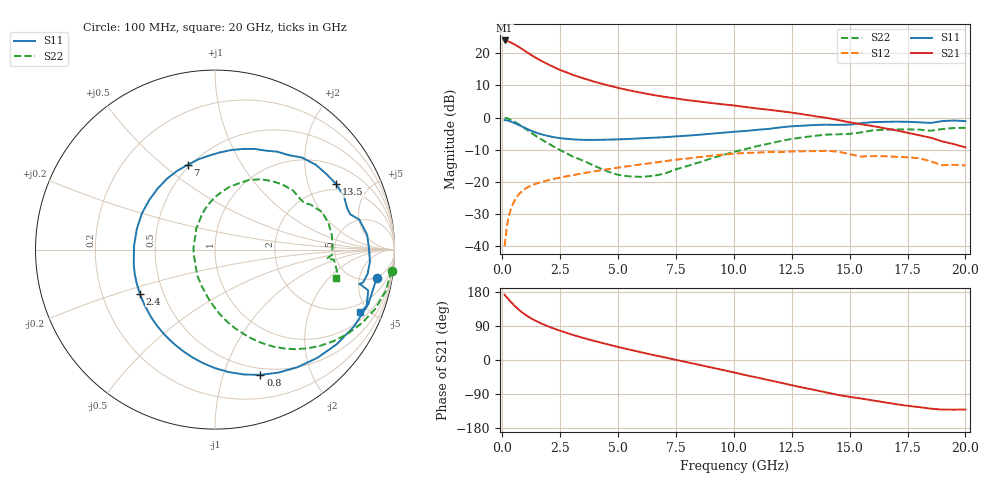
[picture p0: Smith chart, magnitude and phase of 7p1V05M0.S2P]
! Infineon Technologies  Discrete & RF Semiconductors
! bfp620
! VCE =  1.0 V,  IC =  5.0 mA
! Common Emitter S-Parameters:  Sep 2002
# GHz  S  MA  R  50
!  f  S11  S21  S12  S22
! GHz  MAG  ANG  MAG  ANG  MAG  ANG  MAG  ANG
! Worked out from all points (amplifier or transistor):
!   59 points, 100 MHz to 20 GHz, reference 50 ohm
!   highest |S21| = 24.0 dB at 100 MHz (marker M1)
!   |S21| within 3 dB of that: start of sweep to 928.2 MHz
!   unconditionally stable (mu >= 1): 4.888 GHz to 11.5 GHz; 14.86 GHz to 15.22 GHz; 17.01 GHz to end of sweep
!   at 1 GHz: K = 0.32, MSG = 21.3 dB, |S12| = -22.0 dB
!   at 5.5 GHz: K = 1.04, MAG = 10.5 dB, |S12| = -15.0 dB
!   at 20 GHz: K = 1.50, MAG = -1.4 dB, |S12| = -14.8 dB
!   S11 on the Smith chart (normalised r, x): 100 MHz: 5, -9; 800 MHz: 0.43, -1.33; 2.4 GHz: 0.37, -0.24; 7 GHz: 0.49, +0.61; 13.5 GHz: 1.73, +3.07; 20 GHz: 1.40, -4.43
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0.1  0.9147 -9.9  15.77 172.1  0.0101 82.3  0.9912 -6.8
0.2  0.9066 -19.5  15.48 164.9  0.0212 79.8  0.9787 -13.7
0.3  0.8857 -28.8  15.01 157.9  0.0314 74.9  0.9519 -20.3
0.4  0.859 -37.9  14.45 151.2  0.0407 70.1  0.9167 -26.4
0.5  0.83 -46.6  13.84 144.8  0.0492 65.6  0.8771 -32.2
0.6  0.8005 -54.9  13.21 138.9  0.0567 61.5  0.8354 -37.6
0.8  0.7421 -70.1  11.95 128.3  0.0693 54.5  0.7509 -47.2
0.9  0.7137 -77.1  11.33 123.6  0.0744 51.5  0.7098 -51.4
1.1  0.6604 -90.0  10.17 115.3  0.083 46.4  0.6324 -58.8
1.3  0.6145 -101.6  9.135 108.0  0.0898 42.3  0.5638 -65.0
1.5  0.5776 -112.0  8.266 101.7  0.0954 39.1  0.5051 -70.4
1.9  0.5262 -130.0  6.941 90.7  0.105 34.5  0.4137 -79.7
2.4  0.4855 -149.6  5.689 79.1  0.1153 30.2  0.3272 -89.8
3  0.4606 -169.3  4.666 67.1  0.1272 25.9  0.2532 -101.3
3.5  0.4516 177.3  4.074 58.1  0.1372 22.8  0.214 -110.8
5  0.459 142.7  2.899 34.3  0.1674 13.4  0.1294 -149.7
7  0.4964 107.6  2.104 7.1  0.2102 -0.7  0.1347 143.5
8.5  0.5417 87.3  1.778 -12.7  0.2439 -13.5  0.2016 112.4
10.5  0.6202 62.7  1.463 -39.9  0.2821 -34.4  0.3247 83.2
13.5  0.7677 28.3  1.054 -79.2  0.3017 -65.3  0.5213 44.2
17  0.8659 -4.4  0.635 -116.5  0.2469 -95.7  0.6558 7.1
20  0.8825 -23.3  0.346 -130.7  0.181 -110.0  0.6938 -13.0
